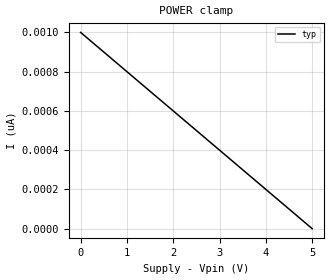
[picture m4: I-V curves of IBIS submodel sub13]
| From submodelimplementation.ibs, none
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| ... this should be also OK
[Submodel] sub13
Submodel_type Dynamic_clamp
[POWER Clamp]
0V        1nA        NA         NA
5V        0A         NA         NA
